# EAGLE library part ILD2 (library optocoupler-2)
SIEMENS OPTO COUPLER
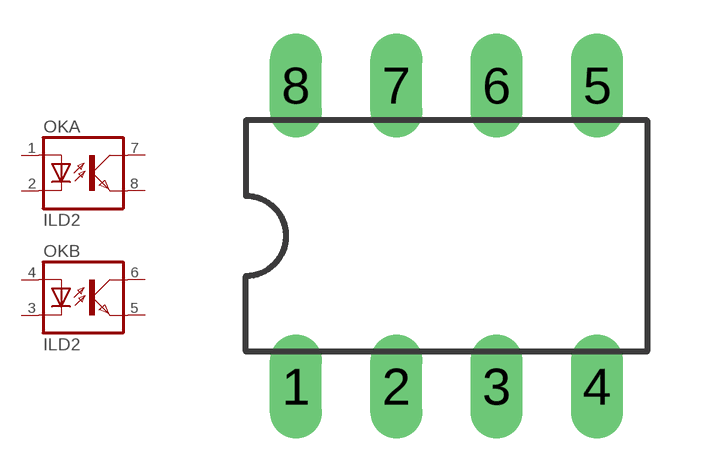
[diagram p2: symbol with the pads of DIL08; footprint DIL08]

Designator prefix OK; gates A=OK B=OK

## ILD2  [DIL08]
1  A:A  pas
2  A:C  pas
3  B:C  pas
4  B:A  pas
5  B:EMIT  pas
6  B:COL  pas
7  A:COL  pas
8  A:EMIT  pas

## Footprint DIL08 (pad centres in mm)
Dual In Line Package
drill 0.813 long: 1 -3.81,-3.81; 2 -1.27,-3.81; 3 1.27,-3.81; 4 3.81,-3.81; 5 3.81,3.81; 6 1.27,3.81; 7 -1.27,3.81; 8 -3.81,3.81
